PROGRAM MAIN
VAR
	fbTp01: TP;
	fbTp02: TP;
	bLed AT%Q*: BOOL;
	fbMC_Power: MC_Power;
	stAxis: AXIS_REF;
	fbMC_MoveAbsolute: MC_MoveAbsolute;
	iState : INT := 100;
	UI_Led AT%MX10.0: BOOL;
	UI_ActPosition: LREAL;
	UI_ActVelocity: LREAL;
	UI_MotorMode: STRING;
	fbMC_Halt: MC_Halt;
	Btn_Stop: BOOL;
	UI_Stop: BOOL;

	fbCtu: CTU;
	iCurrentValue: WORD;
	bEl2008_01 AT%Q*: BOOL;
	bEl2008_02 AT%Q*: BOOL;
	bEl2008_03 AT%Q*: BOOL;
	bEl2008_04 AT%Q*: BOOL;
	bEl2008_05 AT%Q*: BOOL;
	bKl2809_01 AT%Q*: BOOL;
	bKl2809_02 AT%Q*: BOOL;
	bKl2809_03 AT%Q*: BOOL;
	//bKl2809_01 AT%Q*: BOOL;
	
	bManual AT%Q*: BOOL;
	bChDir AT%Q*: BOOL;
	UI_setVelocity: LREAL;
	fbTon: TON;
	fbPowerY: MC_Power;
	stAxisY: AXIS_REF;
	fbMC_MoveVelocity: MC_MoveVelocity;
	bInit: BOOL := true;
	fbMC_SetPosition: MC_SetPosition;
END_VAR

IF bInit THEN
	fbMC_SetPosition(
	Axis:= stAxis, 
	Execute:= TRUE, 
	Position:= 0, 
	Mode:= , 
	Options:= , 
	Done=> , 
	Busy=> , 
	Error=> , 
	ErrorID=> );
	bInit := FALSE;
END_IF

fbTp01(in := NOT fbTp02.Q, pt := T#100MS);
fbTp02(in := NOT fbTp01.Q, pt := T#100MS);

bLed := fbTp01.Q;

fbCtu(
	CU:= fbTp01.Q, 
	RESET:= fbCtu.Q, 
	PV:= 8, 
	Q=> , 
	CV=> iCurrentValue);
	
	CASE iCurrentValue OF
		1:
			bEl2008_01 := TRUE;
			bEl2008_02 := FALSE;
			bEl2008_03 := FALSE;
			bEl2008_04 := FALSE;
			bEl2008_05 := FALSE;
			bKl2809_01 := FALSE;
			bKl2809_02 := FALSE;
			bKl2809_03 := FALSE;
			
		2:
			bEl2008_01 := FALSE;
			bEl2008_02 := TRUE;
			bEl2008_03 := FALSE;
			bEl2008_04 := FALSE;
			bEl2008_05 := FALSE;
			bKl2809_01 := FALSE;
			bKl2809_02 := FALSE;
			bKl2809_03 := FALSE;
			
			3:
			bEl2008_01 := FALSE;
			bEl2008_02 := FALSE;
			bEl2008_03 := TRUE;
			bEl2008_04 := FALSE;
			bEl2008_05 := FALSE;
			bKl2809_01 := FALSE;
			bKl2809_02 := FALSE;
			bKl2809_03 := FALSE;
			
			
			4:
			bEl2008_01 := FALSE;
			bEl2008_02 := FALSE;
			bEl2008_03 := FALSE;
			bEl2008_04 := TRUE;
			bEl2008_05 := FALSE;
			bKl2809_01 := FALSE;
			bKl2809_02 := FALSE;
			bKl2809_03 := FALSE;
			
			5:
			bEl2008_01 := FALSE;
			bEl2008_02 := FALSE;
			bEl2008_03 := FALSE;
			bEl2008_04 := FALSE;
			bEl2008_05 := TRUE;
			bKl2809_01 := FALSE;
			bKl2809_02 := FALSE;
			bKl2809_03 := FALSE;
			
			
		(*	6:
			bEl2008_01 := FALSE;
			bEl2008_02 := FALSE;
			bEl2008_03 := FALSE;
			bEl2008_04 := FALSE;
			bEl2008_05 := FALSE;
			bKl2809_01 := TRUE;
			bKl2809_02 := FALSE;
			bKl2809_03 := FALSE;
			
			
			7:
			bEl2008_01 := FALSE;
			bEl2008_02 := FALSE;
			bEl2008_03 := FALSE;
			bEl2008_04 := FALSE;
			bEl2008_05 := FALSE;
			bKl2809_01 := FALSE;
			bKl2809_02 := TRUE;
			bKl2809_03 := FALSE;
			
			
			8:
			bEl2008_01 := FALSE;
			bEl2008_02 := FALSE;
			bEl2008_03 := FALSE;
			bEl2008_04 := FALSE;
			bEl2008_05 := FALSE;
			bKl2809_01 := FALSE;
			bKl2809_02 := FALSE;
			bKl2809_03 := TRUE;
			*)
			6:
			
			bEl2008_01 := FALSE;
			bEl2008_02 := FALSE;
			bEl2008_03 := FALSE;
			bEl2008_04 := FALSE;
			bEl2008_05 := FALSE;
			bKl2809_01 := FALSE;
			bKl2809_02 := FALSE;
			bKl2809_03 := FALSE;
			
			7:
		
			bEl2008_01 := TRUE;
			bEl2008_02 := TRUE;
			bEl2008_03 := TRUE;
			bEl2008_04 := TRUE;
			bEl2008_05 := TRUE;
			bKl2809_01 := TRUE;
			bKl2809_02 := TRUE;
			bKl2809_03 := TRUE;
	END_CASE


fbMC_Power(
	Axis:= stAxis, 
	Enable:= TRUE, 
	Enable_Positive:= TRUE, 
	Enable_Negative:= TRUE, 
	Override:= 100, 
	BufferMode:= , 
	Options:= , 
	Status=> , 
	Busy=> , 
	Active=> , 
	Error=> , 
	ErrorID=> );
	
	fbMC_MoveAbsolute(
	Axis:= stAxis, 
	Execute:= , 
	Position:= , 
	Velocity:= , 
	Acceleration:= , 
	Deceleration:= , 
	Jerk:= , 
	BufferMode:= , 
	Options:= , 
	Done=> , 
	Busy=> , 
	Active=> , 
	CommandAborted=> , 
	Error=> , 
	ErrorID=> );
	
	
	fbMC_Halt(
	Axis:= stAxis, 
	Execute:= , 
	Deceleration:= , 
	Jerk:= , 
	BufferMode:= , 
	Options:= , 
	Done=> , 
	Busy=> , 
	Active=> , 
	CommandAborted=> , 
	Error=> , 
	ErrorID=> );
	
	
(*	
	IF NOT fbMC_Power.Busy THEN
		IF fbMC_Power.Error THEN
			iState := 99;
			ELSE
				iState := 1;
		END_IF
	END_IF
	*)
	
	
		IF Btn_Stop THEN
		fbMC_Halt.Execute := TRUE;
		ELSE
			fbMC_Halt.Execute := FALSE;
	END_IF
	
	
	CASE iState OF
		100:
			fbTon(in := TRUE, pt := T#2S);
			IF fbTon.Q THEN
				iState := 1;
				fbTon(in := FALSE);	
			END_IF
			
		1:
			fbMC_MoveAbsolute(Axis := stAxis);
		
			fbMC_MoveAbsolute.Velocity := 50;
			fbMC_MoveAbsolute.Position := 20;
			fbMC_MoveAbsolute.Execute := TRUE;
			
			iState := 2;
		
		2:
			fbMC_MoveAbsolute(Axis := stAxis);
			IF NOT fbMC_MoveAbsolute.Busy THEN
				IF fbMC_MoveAbsolute.Error THEN
					iState := 98;
				ELSE
					fbMC_MoveAbsolute.Execute := FALSE;
					iState := 3;
				END_IF
			END_IF
		
		3:
		fbMC_MoveAbsolute(Axis := stAxis);
			fbMC_MoveAbsolute.Velocity := 100;
			fbMC_MoveAbsolute.Position := 100;
			fbMC_MoveAbsolute.Execute := TRUE;
			
			iState := 4;	
			
			4:
			fbMC_MoveAbsolute(Axis := stAxis);
			IF NOT fbMC_MoveAbsolute.Busy THEN
				IF fbMC_MoveAbsolute.Error THEN
					iState := 98;
				ELSE
					fbMC_MoveAbsolute.Execute := FALSE;
					iState := 5;
				END_IF
			END_IF
			
			5:
			fbMC_MoveAbsolute(Axis := stAxis);
			fbMC_MoveAbsolute.Velocity := 100;
			fbMC_MoveAbsolute.Position := 0;
			fbMC_MoveAbsolute.Execute := TRUE;
			
			iState := 6;
			
			6:
			fbMC_MoveAbsolute(Axis := stAxis);
			IF NOT fbMC_MoveAbsolute.Busy THEN
				IF fbMC_MoveAbsolute.Error THEN
					iState := 98;
				ELSE
					fbMC_MoveAbsolute.Execute := FALSE;
					iState := 1;
				END_IF
			END_IF
			
			
		98:
			;// Position error;
			
		99:
			;//Enable Error;	
			
	END_CASE
	

	
	
	
	(************
	
	DATA FOR HMI 
	
	*************)
	
	UI_Led := bLed;
	
	UI_ActPosition := stAxis.NcToPlc.ActPos;
	UI_ActVelocity := stAxis.NcToPlc.ActVelo;
	Btn_Stop := UI_Stop; 
	
	IF iState = 2 OR iState = 4 THEN
		UI_MotorMode := 'FORWARDING';
		ELSIF iState = 6 THEN
			UI_MotorMode := 'BACKWARDING';
			ELSE
				UI_MotorMode := 'STOPPING';
	
	END_IF
	
	
	fbPowerY(
	Axis:= stAxisY, 
	Enable:= TRUE, 
	Enable_Positive:= TRUE, 
	Enable_Negative:= TRUE, 
	Override:= 100, 
	BufferMode:= , 
	Options:= , 
	Status=> , 
	Busy=> , 
	Active=> , 
	Error=> , 
	ErrorID=> );
	
	
	IF fbPowerY.Status THEN
	fbMC_MoveVelocity(
	Axis:= stAxisY, 
	Execute:= TRUE, 
	Velocity:= 10, 
	Acceleration:= , 
	Deceleration:= , 
	Jerk:= , 
	Direction:= , 
	BufferMode:= , 
	Options:= , 
	InVelocity=> , 
	Busy=> , 
	Active=> , 
	CommandAborted=> , 
	Error=> , 
	ErrorID=> );
	END_IF

END_PROGRAM
